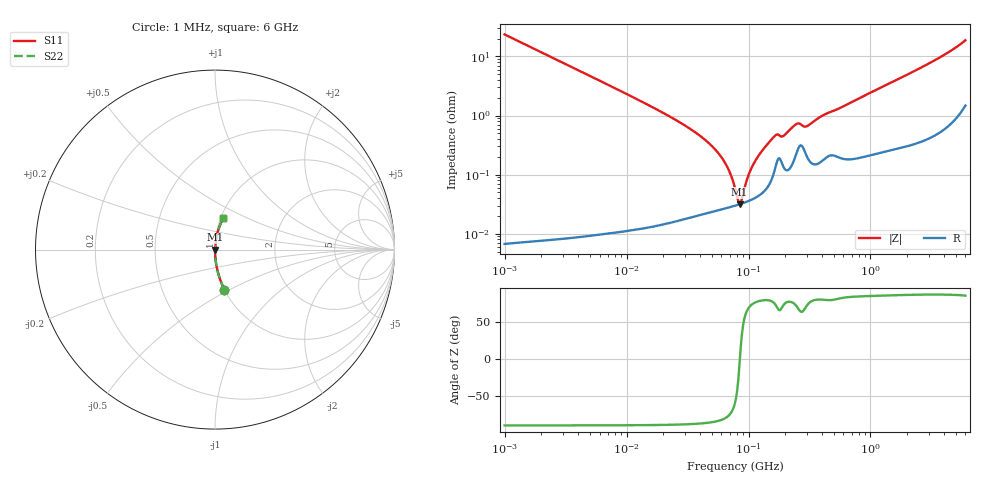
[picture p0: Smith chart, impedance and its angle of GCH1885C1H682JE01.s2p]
!Murata Part Number: GCH1885C1H682JE01
!These Parameters are Measured in Series Mode Connection
!Data Generated on Jun 19, 2026
!  o--ll--o
!Port1  Port2
!  o------o
!Operation Temp=25[degC], DC Bias Voltage=0[V]
!Freq. Start=1000[kHz] Stop=6[GHz] 401[Steps]
# Hz S RI R 50
!Freq.(Hz) S11(Real) S11(Imag) S21(Real) S21(Imag) S12(Real) S12(Imag) S22(Real) S22(Imag)
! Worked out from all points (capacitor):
!   401 points, 1 MHz to 6 GHz, reference 50 ohm
!   read as one part in series: C = 6.76 nF near 1.044 MHz
!   lowest |Z| = 31.7 mohm at 84.5 MHz (marker M1)
!   series resonance near 84.95 MHz, so ESL is about 520 pH
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1000000  0.0525 -0.2229  0.9475 0.2229  0.9475 0.2229  0.0525 -0.2229
4293785  0.00307 -0.0545  0.9969 0.0545  0.9969 0.0545  0.00307 -0.0545
1.843659e7  0.000285 -0.0121  0.9997 0.0121  0.9997 0.0121  0.000285 -0.0121
3.46415e7  0.000223 -0.00562  0.9998 0.00562  0.9998 0.00562  0.000223 -0.00562
5.124051e7  0.000245 -0.00289  0.9998 0.00289  0.9998 0.00289  0.000245 -0.00289
6.652088e7  0.000275 -0.00136  0.9997 0.00136  0.9997 0.00136  0.000275 -0.00136
7.256705e7  0.000288 -0.000871  0.9997 0.000871  0.9997 0.000871  0.000288 -0.000871
7.745967e7  0.000298 -0.00051  0.9997 0.00051  0.9997 0.00051  0.000298 -0.00051
8.090333e7  0.000307 -0.000269  0.9997 0.000269  0.9997 0.000269  0.000307 -0.000269
8.450008e7  0.000315 -2.9e-05  0.9997 2.9e-05  0.9997 2.9e-05  0.000315 -2.9e-05
8.825674e7  0.000325 0.000212  0.9997 -0.000212  0.9997 -0.000212  0.000325 0.000212
9.83954e7  0.000354 0.000823  0.9996 -0.000823  0.9996 -0.000823  0.000354 0.000823
1.096987e8  0.000392 0.00146  0.9996 -0.00146  0.9996 -0.00146  0.000392 0.00146
1.587717e8  0.000977 0.00409  0.999 -0.00409  0.999 -0.00409  0.000977 0.00409
1.694764e8  0.00156 0.00448  0.9984 -0.00448  0.9984 -0.00448  0.00156 0.00448
1.930997e8  0.00138 0.00429  0.9986 -0.00429  0.9986 -0.00429  0.00138 0.00429
2.506837e8  0.00253 0.00683  0.9975 -0.00683  0.9975 -0.00683  0.00253 0.00683
2.919064e8  0.00238 0.006  0.9976 -0.006  0.9976 -0.006  0.00238 0.006
3.325952e8  0.00159 0.00744  0.9984 -0.00744  0.9984 -0.00744  0.00159 0.00744
1.428092e9  0.00373 0.0346  0.9963 -0.0346  0.9963 -0.0346  0.00373 0.0346
3.408564e9  0.0121 0.0858  0.9879 -0.0858  0.9879 -0.0858  0.0121 0.0858
6e9  0.047 0.1759  0.953 -0.1759  0.953 -0.1759  0.047 0.1759
